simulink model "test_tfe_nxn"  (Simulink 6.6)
settings: Solver=ode45  StartTime=0.0  StopTime=10.0  RelTol=1e-3
undefined symbols (not defined in the file or in its folder): Generator, test_tfe_nxn
libraries: sltpda x14

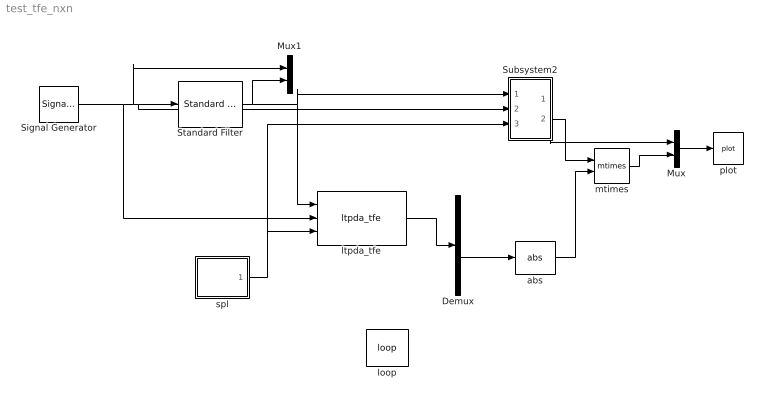
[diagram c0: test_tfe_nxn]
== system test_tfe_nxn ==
  Demux : Demux
  Mux : Mux  Inputs=2
  Mux1 : Mux  Inputs=2
  Signal Generator : sltpda/Sources/Signal Generator  Tag=ao  SystemSampleTime=-1  nsecs=10  fs=100  tsfcn=randn(size(t))
  Standard Filter : sltpda/Signal Processing blocks/Digital filtering/Standard Filter  Tag=filter  Description=Apply a standard filter type to input AO.  SystemSampleTime=-1  method=filter  ftype=highpass  fgain=1  ffc=10  forder=1
  Subsystem2 : Subsystem
  abs : sltpda/math blocks/abs  SystemSampleTime=-1
  loop : sltpda/Parameters/loop  SystemSampleTime=-1  block=test_tfe_nxn/Signal Generator  blockHandle=170.0015869140625  key=nsecs  vals=10 20 30  loopon=on
  ltpda_tfe : sltpda/Signal Processing blocks/Frequency domain/ltpda_tfe  Tag=ltpda_tfe  Description=Calls ltpda_tfe.  SystemSampleTime=-1  win=Hanning  nfft=200
  mtimes : sltpda/math blocks/mtimes  Tag=mtimes  SystemSampleTime=-1
  plot : sltpda/Sinks/plot  Tag=plot  Description=Plot an analysis object.  SystemSampleTime=-1  xscale=linear  yscale=linear
  spl : Subsystem
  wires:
  Signal Generator/1 -> ltpda_tfe/2, Standard Filter/1, Subsystem2/2(In2), Mux1/1
  Standard Filter/1 -> ltpda_tfe/1, Subsystem2/1(In1), Mux1/2
  ltpda_tfe/1 -> Demux/1
  Subsystem2/2(Out2) -> mtimes/1
  Demux/3 -> abs/1
  abs/1 -> mtimes/2
  Subsystem2/1(Out1) -> Mux/1
  mtimes/1 -> Mux/2
  Mux/1 -> plot/1
  spl/1(Out1) -> ltpda_tfe/3, Subsystem2/3(In3)

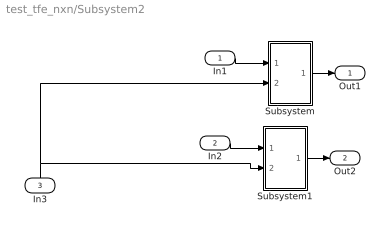
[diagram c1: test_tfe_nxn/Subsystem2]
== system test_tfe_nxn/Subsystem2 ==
  In1 : Inport
  In2 : Inport  Port=2
  In3 : Inport  Orientation=up  Port=3
  Subsystem : Subsystem
  Subsystem1 : Subsystem
  Out1 : Outport
  Out2 : Outport  Port=2
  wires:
  In1/1 -> Subsystem/1(In1)
  In2/1 -> Subsystem1/1(In1)
  In3/1 -> Subsystem/2(In2), Subsystem1/2(In2)
  Subsystem/1(Out1) -> Out1/1
  Subsystem1/1(Out1) -> Out2/1

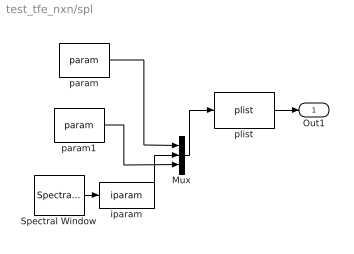
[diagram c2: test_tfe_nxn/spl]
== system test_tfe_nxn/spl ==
  Mux : Mux  Inputs=3
  Spectral Window : sltpda/Sources/Spectral Window  Tag=specwin  SystemSampleTime=-1  wname=Kaiser  wlen=50  psll=100
  iparam : sltpda/Parameters/iparam  Tag=iparam  SystemSampleTime=-1  key=Win
  param : sltpda/Parameters/param  Tag=param  SystemSampleTime=-1  key=Nfft  val=0
  param1 : sltpda/Parameters/param  Tag=param  SystemSampleTime=-1  key=Nolap  val=0
  plist : sltpda/Parameters/plist  SystemSampleTime=-1
  Out1 : Outport
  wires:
  plist/1 -> Out1/1
  iparam/1 -> Mux/2
  Spectral Window/1 -> iparam/1
  param/1 -> Mux/1
  Mux/1 -> plist/1
  param1/1 -> Mux/3

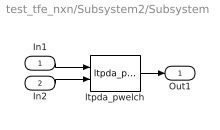
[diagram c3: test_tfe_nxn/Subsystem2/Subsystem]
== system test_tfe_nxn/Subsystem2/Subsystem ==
  In1 : Inport
  In2 : Inport  Port=2
  ltpda_pwelch : sltpda/Signal Processing blocks/Frequency domain/ltpda_pwelch  Tag=ltpda_pwelch  Description=Makes a spectral density estimate by calling ltpda_pwlech.  SystemSampleTime=-1  Nfft=200  Nolap=-1
  Out1 : Outport
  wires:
  In1/1 -> ltpda_pwelch/1
  In2/1 -> ltpda_pwelch/2
  ltpda_pwelch/1 -> Out1/1

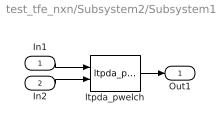
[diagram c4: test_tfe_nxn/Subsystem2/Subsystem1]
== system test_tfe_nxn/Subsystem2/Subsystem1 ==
  In1 : Inport
  In2 : Inport  Port=2
  ltpda_pwelch : sltpda/Signal Processing blocks/Frequency domain/ltpda_pwelch  Tag=ltpda_pwelch  Description=Makes a spectral density estimate by calling ltpda_pwlech.  SystemSampleTime=-1  Nfft=200  Nolap=-1
  Out1 : Outport
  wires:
  In1/1 -> ltpda_pwelch/1
  In2/1 -> ltpda_pwelch/2
  ltpda_pwelch/1 -> Out1/1
